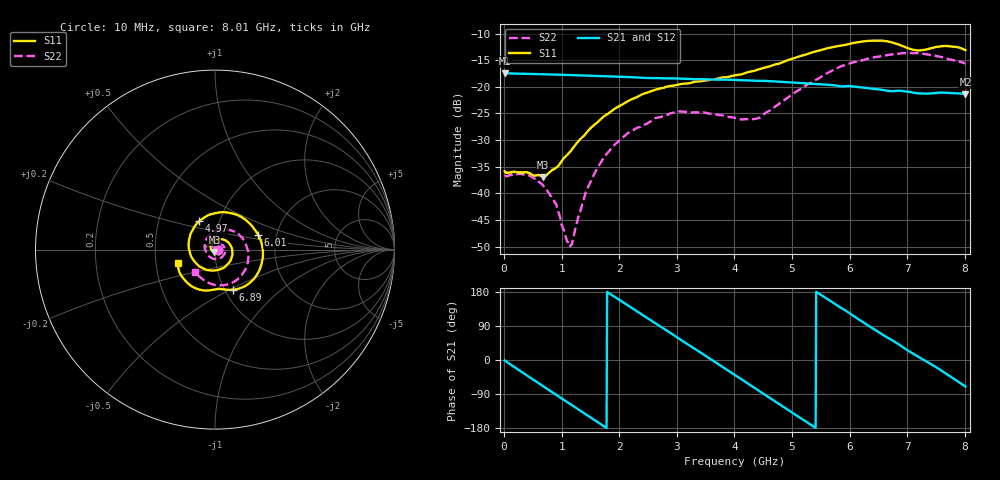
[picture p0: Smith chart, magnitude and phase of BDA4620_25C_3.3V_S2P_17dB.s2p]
!Agilent Technologies,E5071B,MY42404982,A.09.10
!Date: Wed May 06 08:52:17 2026
!Data & Calibration Information:
!Freq	S11:SOLT2(ON)	S21:SOLT2(ON)	S12:SOLT2(ON)	S22:SOLT2(ON)
# Hz S RI R 50
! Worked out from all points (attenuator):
!   801 points, 10 MHz to 8.01 GHz, reference 50 ohm
!   highest |S21| = -17.42 dB at 10 MHz (marker M1); lowest = -21.4 dB at 8.01 GHz (marker M2)
!   lowest |S11| = -36.9 dB at 680 MHz (marker M3), VSWR 1.03, Z = 49.7 - j1.38 ohm
!   |S11| at or under -10 dB: start of sweep to end of sweep
!   |S22| runs from -49.9 to -13.6 dB; largest |S21 - S12| = 0.00065
!   S11 on the Smith chart (normalised r, x): 10 MHz: 1.03, -0.00; 4.97 GHz: 0.80, +0.26; 6.01 GHz: 1.60, +0.28; 6.89 GHz: 1.09, -0.52; 8.01 GHz: 0.65, -0.11
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1e7  0.0161 -0.00113  0.1346 -0.00287  0.1347 -0.00291  0.0145 -0.000534
4.3e8  0.00848 -0.0131  0.0953 -0.092  0.0954 -0.0923  0.0136 -0.00575
6.8e8  -0.00326 -0.0139  0.0466 -0.1229  0.0465 -0.1231  0.00892 -0.00771
8.9e8  -0.0147 -0.00895  -0.000956 -0.1304  -0.00106 -0.1306  0.00325 -0.00747
1.14e9  -0.0235 0.0062  -0.0557 -0.1166  -0.056 -0.1168  -0.00276 -0.00185
1.19e9  -0.0242 0.0104  -0.0656 -0.1109  -0.0657 -0.1111  -0.00359 -6.13e-05
1.35e9  -0.0237 0.0234  -0.0931 -0.088  -0.0932 -0.088  -0.00527 0.00544
1.58e9  -0.0136 0.0422  -0.1188 -0.0443  -0.119 -0.0444  -0.00432 0.0151
1.87e9  0.0131 0.0577  -0.1239 0.0183  -0.1241 0.0184  0.00408 0.0263
2.68e9  0.0956 0.000922  -0.00361 0.1208  -0.00349 0.1209  0.0478 0.0192
3.41e9  0.0341 -0.1074  0.1111 0.0401  0.1113 0.04  0.0446 -0.0365
4.01e9  -0.0937 -0.0878  0.0893 -0.0745  0.0893 -0.0747  -0.0145 -0.0492
4.42e9  -0.1459 0.0074  0.0187 -0.1126  0.0186 -0.1127  -0.0497 -0.0122
4.97e9  -0.0882 0.1584  -0.0788 -0.0772  -0.0789 -0.0772  -0.037 0.0738
5.35e9  0.0334 0.2084  -0.1061 -0.0127  -0.1062 -0.0126  0.0246 0.1081
6.01e9  0.241 0.0816  -0.0539 0.0862  -0.0541 0.0864  0.1555 0.0606
6.35e9  0.2631 -0.0647  0.00277 0.0966  0.00275 0.0967  0.1848 -0.0143
6.68e9  0.1825 -0.1939  0.0497 0.0766  0.0499 0.0768  0.1741 -0.0978
6.89e9  0.1006 -0.2242  0.073 0.0558  0.0732 0.0559  0.1466 -0.1455
7.19e9  0.0191 -0.2187  0.0858 0.0135  0.086 0.0137  0.0758 -0.1927
7.56e9  -0.0925 -0.2207  0.0802 -0.0368  0.0804 -0.0369  -0.0218 -0.1906
8.01e9  -0.2078 -0.0771  0.0295 -0.0802  0.0296 -0.0803  -0.1101 -0.1238
